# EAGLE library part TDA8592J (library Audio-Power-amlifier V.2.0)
The TDA8592J is a complementary quad BTL audio power amplifier made in BCDMOS technology. It contains four independent amplifiers in Bridge Tied Load (BTL) configuration. Through the I2C-bus, the diagnostic information of each amplifier and speaker can be read separately
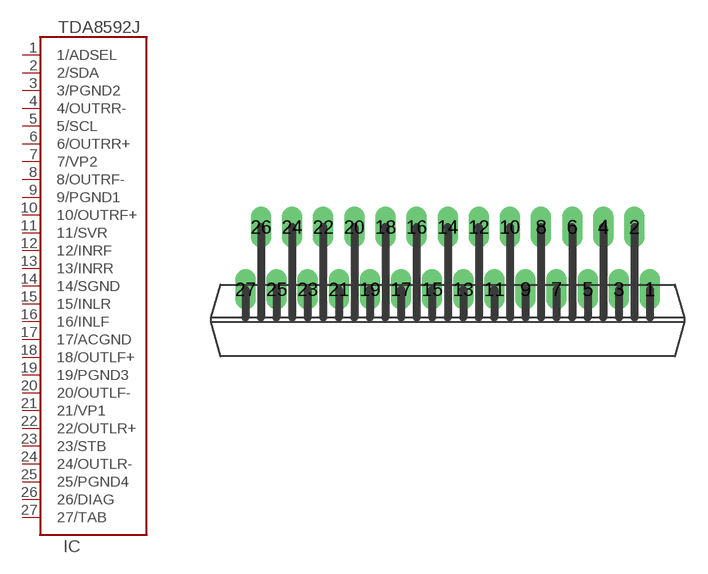
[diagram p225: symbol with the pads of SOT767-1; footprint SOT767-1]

Designator prefix IC

## TDA8592J  [SOT767-1]
1  1/ADSEL
2  2/SDA
3  3/PGND2  pwr
4  4/OUTRR-  out
5  5/SCL  in
6  6/OUTRR+  out
7  7/VP2  pwr
8  8/OUTRF-  out
9  9/PGND1  pwr
10  10/OUTRF+  out
11  11/SVR
12  12/INRF  in
13  13/INRR  in
14  14/SGND  pwr
15  15/INLR  in
16  16/INLF  in
17  17/ACGND  pwr
18  18/OUTLF+  out
19  19/PGND3  pwr
20  20/OUTLF-  out
21  21/VP1  pwr
22  22/OUTLR+  out
23  23/STB  in
24  24/OUTLR-  out
25  25/PGND4  pwr
26  26/DIAG  out
27  27/TAB

## Footprint SOT767-1 (pad centres in mm)
drill 0.8 long: 1 13,0; 2 12,4; 3 11,0; 4 10,4; 5 9,0; 6 8,4; 7 7,0; 8 6,4; 9 5,0; 10 4,4; 11 3,0; 12 2,4; 13 1,0; 14 0,4; 15 -1,0; 16 -2,4; 17 -3,0; 18 -4,4; 19 -5,0; 20 -6,4; 21 -7,0; 22 -8,4; 23 -9,0; 24 -10,4; 25 -11,0; 26 -12,4; 27 -13,0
